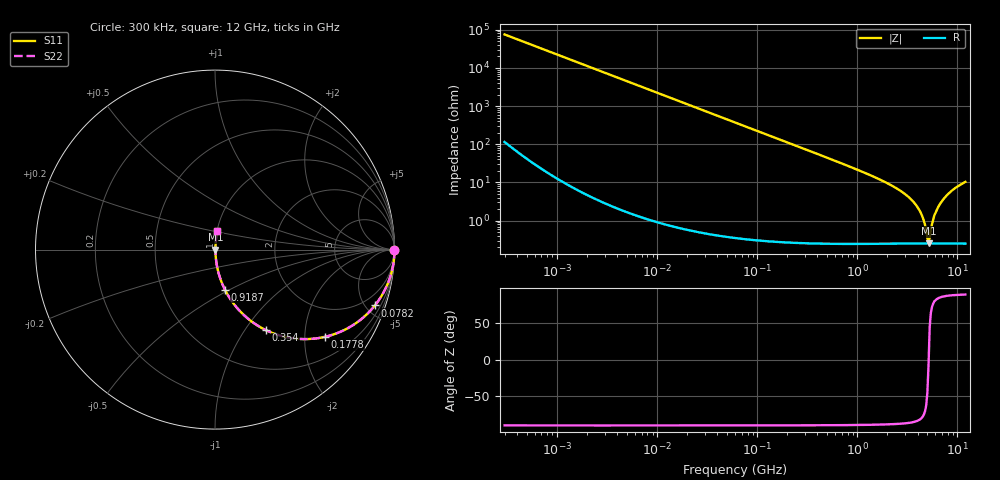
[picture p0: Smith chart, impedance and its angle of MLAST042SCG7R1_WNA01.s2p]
! MLAST042SCG7R1_WNA01  S-PARAMETER MODEL  ( General Type )
! Model Generated by TAIYO YUDEN Corporation (http://www.ty-top.com)
! Version 1.0
! TAIYO YUDEN Control No. 150820
! Copyright(c) 2015 TAIYO YUDEN CO.,LTD. All Rights Reserved.
! Product Description (link to TY-COMPAS)
! https://ds.yuden.co.jp/TYCOMPAS/or/detail?pn=MLAST042SCG7R1BWNA01&u=M
! Products Name : Multilayer Ceramic Capacitors
! Characteristics :
!  Capacitance : 7.1 pF , Rated Voltage : 25V , TCC : CG / C0G
!  Case Size : 0.4 x 0.2 / 0.016 x 0.008 [mm/inch] , Thickness : 0.2 / 0.008 [mm/inch]
!  (Conditions: Temperature = 25 degC , DC Bias Current/Voltage = 0A / 0V)
! External Node Assignments :
!  1  o---| |---o  2
! GND o---------o GND
! Frequency Range : 0.3MHz  -  12000MHz  [ 401 STEP ]
# MHz S RI R 50
! Freq[MHz].  S11 Real  S11 Imag  S21 Real  S21 Imag  S12 Real  S12 Imag  S22 Real  S22 Imag
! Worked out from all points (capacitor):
!   401 points, 300 kHz to 12 GHz, reference 50 ohm
!   read as one part in series: C = 7.11 pF near 316.3 kHz
!   lowest |Z| = 256 mohm at 5.141 GHz (marker M1)
!   series resonance near 5.157 GHz, so ESL is about 130 pH
!   S11 on the Smith chart (normalised r, x): 300 kHz: open; 78.2 MHz: 1.01, -5.72; 177.8 MHz: 1.01, -2.52; 354 MHz: 1.01, -1.26; 918.7 MHz: 1.00, -0.47; 12 GHz: 1.01, +0.21
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0.3  1 -0.00134  3.85e-06 0.00134  3.85e-06 0.00134  1 -0.00134
1.769972  0.9999 -0.00791  6.59e-05 0.00791  6.59e-05 0.00791  0.9999 -0.00791
10.44266  0.9978 -0.0465  0.00219 0.0465  0.00219 0.0465  0.9978 -0.0465
27.10171  0.9855 -0.1193  0.0145 0.1193  0.0145 0.1193  0.9855 -0.1193
60  0.9328 -0.2499  0.0672 0.2499  0.0672 0.2499  0.9328 -0.2499
78.19928  0.8909 -0.3111  0.1091 0.3111  0.1091 0.3111  0.8909 -0.3111
177.7716  0.6125 -0.4861  0.3875 0.4861  0.3875 0.4861  0.6125 -0.4861
353.9943  0.2846 -0.4492  0.7154 0.4492  0.7154 0.4492  0.2846 -0.4492
918.7169  0.0548 -0.2225  0.9452 0.2225  0.9452 0.2225  0.0548 -0.2225
2088.533  0.0104 -0.0885  0.9896 0.0885  0.9896 0.0885  0.0104 -0.0885
3026.31  0.00484 -0.0481  0.9952 0.0481  0.9952 0.0481  0.00484 -0.0481
3841.137  0.00319 -0.0258  0.9968 0.0258  0.9968 0.0258  0.00319 -0.0258
4385.161  0.00273 -0.014  0.9973 0.014  0.9973 0.014  0.00273 -0.014
4623.766  0.00262 -0.00942  0.9974 0.00942  0.9974 0.00942  0.00262 -0.00942
4875.354  0.00255 -0.00483  0.9974 0.00483  0.9974 0.00483  0.00255 -0.00483
5140.631  0.00253 -0.000335  0.9975 0.000335  0.9975 0.000335  0.00253 -0.000335
5420.343  0.00256 0.00507  0.9974 -0.00507  0.9974 -0.00507  0.00256 0.00507
5715.274  0.00264 0.0102  0.9974 -0.0102  0.9974 -0.0102  0.00264 0.0102
6026.253  0.00278 0.0157  0.9972 -0.0157  0.9972 -0.0157  0.00278 0.0157
6879.757  0.00344 0.0301  0.9966 -0.0301  0.9966 -0.0301  0.00344 0.0301
8732.115  0.0061 0.0596  0.9939 -0.0596  0.9939 -0.0596  0.0061 0.0596
12000  0.0131 0.1022  0.9869 -0.1022  0.9869 -0.1022  0.0131 0.1022
